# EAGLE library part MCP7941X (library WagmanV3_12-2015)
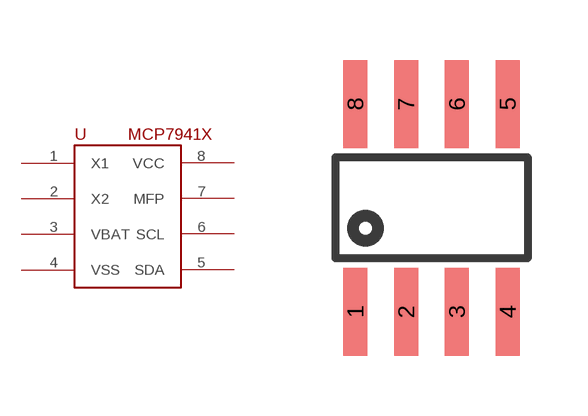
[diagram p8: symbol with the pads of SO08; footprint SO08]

Designator prefix U

## MCP7941X-SOIC-8  [SO08]
1  X1  pas
2  X2  pas
3  VBAT  pas
4  VSS  pas
5  SDA  pas
6  SCL  pas
7  MFP  pas
8  VCC  pas

## Footprint SO08 (pad centres in mm)
SMALL OUTLINE INTEGRATED CIRCUIT body 3.9 mm/JEDEC MS-012AA
smd 0.6 x 2.2: 1 -1.905,-2.6; 2 -0.635,-2.6; 3 0.635,-2.6; 4 1.905,-2.6; 5 1.905,2.6; 6 0.635,2.6; 7 -0.635,2.6; 8 -1.905,2.6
